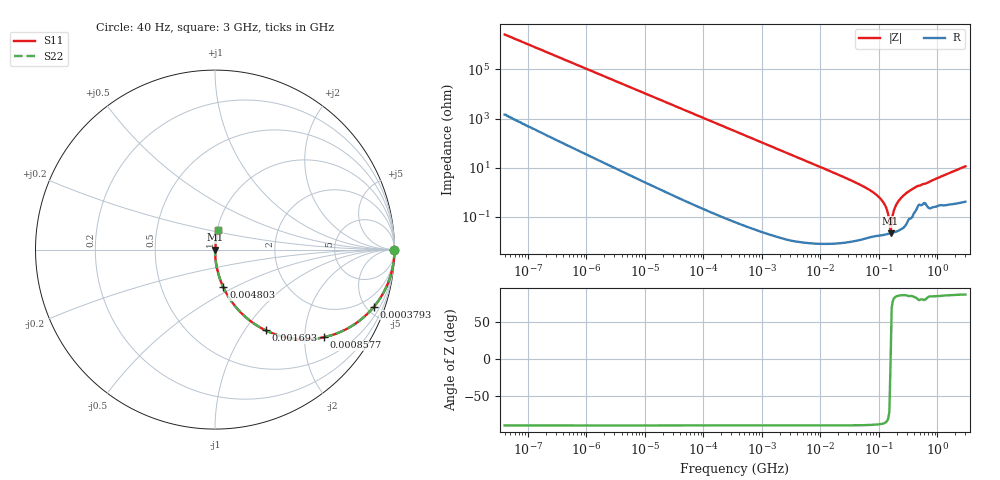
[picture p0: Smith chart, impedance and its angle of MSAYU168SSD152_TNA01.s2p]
! MSAYU168SSD152_TNA01  S-PARAMETER MODEL  ( General Type )
! Model Generated by TAIYO YUDEN Corporation (http://www.ty-top.com)
! Version 3.0
! TAIYO YUDEN Control No. 160201
! Copyright(c) 2003 TAIYO YUDEN CO.,LTD. All Rights Reserved.
! Product Description (link to TY-COMPAS)
! https://ds.yuden.co.jp/TYCOMPAS/or/detail?pn=MSAYU168SSD152KTNA01&u=M
! Products Name : Multilayer Ceramic Capacitors
! Characteristics :
!  Capacitance : 1500 pF , Rated Voltage : 50V
!  Case Size : 1.6 x 0.8 / 0.063 x 0.031 [mm/inch] , Thickness : 0.8 / 0.031 [mm/inch]
!  (Conditions: Temperature = 25 degC , DC Bias Current/Voltage = 0A / 0V)
! External Node Assignments :
!  1  o---| |---o  2
! GND o---------o GND
! Frequency Range : 0.00004MHz  -  3000MHz  [ 401 STEP ]
# MHz S RI R 50
! Freq[MHz].  S11 Real  S11 Imag  S21 Real  S21 Imag  S12 Real  S12 Imag  S22 Real  S22 Imag
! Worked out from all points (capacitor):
!   401 points, 40 Hz to 3 GHz, reference 50 ohm
!   read as one part in series: C = 1.5 nF near 44 Hz
!   lowest |Z| = 21.4 mohm at 157.6 MHz (marker M1)
!   series resonance near 157.9 MHz, so ESL is about 680 pH
!   S11 on the Smith chart (normalised r, x): 40 Hz: open; 379.3 kHz: 1.00, -5.59; 857.7 kHz: 1.00, -2.47; 1.693 MHz: 1.00, -1.25; 4.803 MHz: 1.00, -0.44; 3 GHz: 1.01, +0.23
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4e-05  1 -3.77e-05  2.2e-08 3.77e-05  2.2e-08 3.77e-05  1 -3.77e-05
0.000108  1 -0.000102  5.7e-08 0.000102  5.7e-08 0.000102  1 -0.000102
0.000834  1 -0.000786  8.8e-07 0.000786  8.8e-07 0.000786  1 -0.000786
0.017386  0.9997 -0.0164  0.000272 0.0164  0.000272 0.0164  0.9997 -0.0164
0.101865  0.9908 -0.0952  0.00916 0.0952  0.00916 0.0952  0.9908 -0.0952
0.362475  0.8953 -0.306  0.1047 0.306  0.1047 0.306  0.8953 -0.306
0.379285  0.8865 -0.3171  0.1135 0.3171  0.1135 0.3171  0.8865 -0.3171
0.857716  0.6045 -0.4888  0.3955 0.4888  0.3955 0.4888  0.6045 -0.4888
1.693006  0.2818 -0.4497  0.7182 0.4497  0.7182 0.4497  0.2818 -0.4497
4.802579  0.0465 -0.2103  0.9535 0.2103  0.9535 0.2103  0.0465 -0.2103
7.222098  0.0211 -0.1434  0.9789 0.1434  0.9789 0.1434  0.0211 -0.1434
36.93337  0.000835 -0.0271  0.9992 0.0271  0.9992 0.0271  0.000835 -0.0271
79.8195  0.000254 -0.00986  0.9997 0.00986  0.9997 0.00986  0.000254 -0.00986
120.0322  0.000196 -0.00371  0.9998 0.00371  0.9998 0.00371  0.000196 -0.00371
131.4235  0.000197 -0.00247  0.9998 0.00247  0.9998 0.00247  0.000197 -0.00247
150.5692  0.000207 -0.000626  0.9998 0.000626  0.9998 0.000626  0.000207 -0.000626
157.552  0.000213 -2.57e-05  0.9998 2.57e-05  0.9998 2.57e-05  0.000213 -2.57e-05
172.504  0.000227 0.0012  0.9998 -0.0012  0.9998 -0.0012  0.000227 0.0012
188.875  0.000247 0.00245  0.9998 -0.00245  0.9998 -0.00245  0.000247 0.00245
206.7996  0.000273 0.00371  0.9997 -0.00371  0.9997 -0.00371  0.000273 0.00371
310.9844  0.000762 0.0102  0.9992 -0.0102  0.9992 -0.0102  0.000762 0.0102
3000  0.0166 0.1109  0.9834 -0.1109  0.9834 -0.1109  0.0166 0.1109
